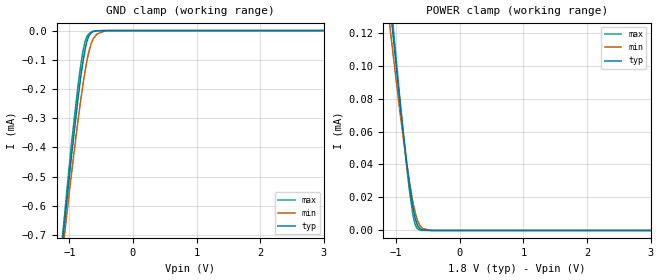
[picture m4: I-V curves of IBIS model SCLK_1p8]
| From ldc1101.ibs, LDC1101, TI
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|   Model
[Model]   SCLK_1p8
Model_type   Input
Vinl = 0.54
Vinh = 1.26
|   typ   min   max
C_comp   0.346pF   0.312pF   0.398pF
[Voltage Range]   1.8   1.71   1.89
[Temperature Range]   27   125   -40
[Power Clamp Reference]   1.8   1.71   1.89
[GND Clamp Reference]   0   0   0
[GND Clamp]
|   Voltage   I(typ)   I(min)   I(max)
-1.8V     -2.267mA   -2.161mA   -2.385mA
-1.141V   -800.1uA   -825.9uA   -783.8uA
-984.6mV  -470.6uA   -526.3uA   -430.2uA
-865.8mV  -239.7uA   -313.8uA   -196.1uA
-811.8mV  -147.6uA   -225.6uA   -107.8uA
-784.8mV  -107.2uA   -184.9uA   -71.08uA
-752.4mV  -66.16uA   -140uA     -38.2uA
-693mV    -19.54uA   -73.65uA   -11.45uA
-655.2mV  -7.821uA   -44.95uA   -5.387uA
-568.8mV  -885.8nA   -12.18uA   -536.5nA
-412.2mV  -5.557nA   -448.9nA   0A
3.6V      0A         0A         0A
[POWER Clamp]
|   Voltage   I(typ)   I(min)   I(max)
-1.8V     418.3uA    371.1uA    454.7uA
-1.12V    145.3uA    130.5uA    154.4uA
-973.8mV  90.14uA    82.59uA    93.21uA
-876.6mV  55.53uA    52.87uA    54.61uA
-833.4mV  41.23uA    40.66uA    38.65uA
-795.6mV  29.64uA    30.75uA    25.82uA
-741.6mV  15.45uA    18.4uA     10.78uA
-698.4mV  7.226uA    10.64uA    3.492uA
-655.2mV  2.575uA    5.279uA    749.9nA
-579.6mV  268.7nA    1.106uA    32.45nA
-439.2mV  0A         34.99nA    0A
3.6V      0A         0A         0A
